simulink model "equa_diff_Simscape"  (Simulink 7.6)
settings: Solver=ode15s  StartTime=0.0  StopTime=30  RelTol=1e-3
InitFcn:
  | w0=0.5; z=sqrt(2)/2;
StopFcn:
  | close all
  | load equa_diff_RLC.mat
  | plot(x(1,:),x(2,:),x(1,:),x(3,:))
  | grid
  | axis([0 30 0 1.2])
  | title('entrée et tension aux bornes de la capacité - RLC')
  | xlabel('temps')
libraries: fl_lib x6, nesl_utility x3

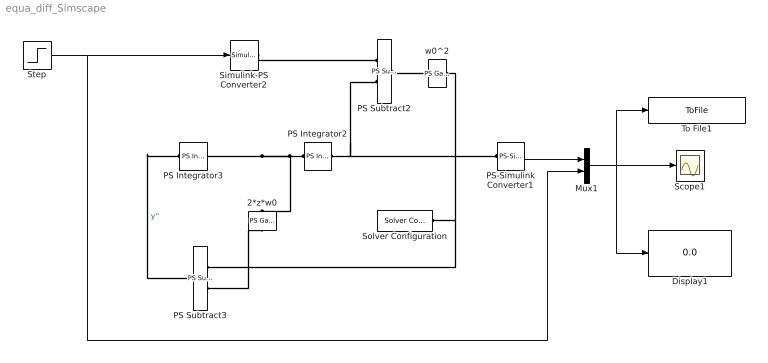
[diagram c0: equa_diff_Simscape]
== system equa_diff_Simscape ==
  2*z*w0 : fl_lib/Physical Signals/Functions/PS Gain  DialogController=NetworkEngine.DynNeDlgSource  SystemSampleTime=-1  gain=2*z*w0  LocalVarLogging=[]
  Display1 : Display
  Mux1 : Mux  Inputs=2
  PS Integrator2 : fl_lib/Physical Signals/Linear Operators/PS Integrator  DialogController=NetworkEngine.DynNeDlgSource  SystemSampleTime=-1  x0=0  x_Log=off  LocalVarNames=|x  LocalVarDescs=|x  LocalVarLogging=0
  PS Integrator3 : fl_lib/Physical Signals/Linear Operators/PS Integrator  DialogController=NetworkEngine.DynNeDlgSource  SystemSampleTime=-1  x0=0  x_Log=off  LocalVarNames=|x  LocalVarDescs=|x  LocalVarLogging=0
  PS Subtract2 : fl_lib/Physical Signals/Functions/PS Subtract  DialogController=NetworkEngine.DynNeDlgSource  SystemSampleTime=-1  LocalVarLogging=[]
  PS Subtract3 : fl_lib/Physical Signals/Functions/PS Subtract  DialogController=NetworkEngine.DynNeDlgSource  SystemSampleTime=-1  LocalVarLogging=[]
  PS-Simulink Converter1 : nesl_utility/PS-Simulink Converter  DialogController=NetworkEngine.DynNeUtilDlgSource  SystemSampleTime=-1  PhysicalDomain=network_engine_domain  LeftPortType=input  RightPortType=output  SubClassName=ps_output  Unit=1  AffineConversion=off
  Scope1 : Scope
  Simulink-PS Converter2 : nesl_utility/Simulink-PS Converter  DialogController=NetworkEngine.DynNeUtilDlgSource  SystemSampleTime=-1  PhysicalDomain=network_engine_domain  LeftPortType=input  RightPortType=output  SubClassName=ps_input  Unit=1  AffineConversion=off  InputFilterTimeConstant=.001  UdotUserProvided=0
  Solver Configuration : nesl_utility/Solver Configuration  DialogController=NetworkEngine.DynNeUtilDlgSource  SystemSampleTime=-1  PhysicalDomain=network_engine_domain  LeftPortType=input  RightPortType=generic  SubClassName=solver  Accelerate=off  Profile=off  ResidualTolerance=1e-9  MaxNonlinIter=3  MaxModeIter=2  DoFixedCost=off  UseLocalSampling=off  DoDC=off  LinearAlgebra=Sparse  LocalSolverSampleTime=.001  LocalSolverChoice=NE_BACKWARD_EULER_ADVANCER  UseLocalSolver=off
  Step : Step  Time=5  SampleTime=0
  To File1 : ToFile  Filename=equa_diff_RLC  MatrixName=x
  w0^2 : fl_lib/Physical Signals/Functions/PS Gain  DialogController=NetworkEngine.DynNeDlgSource  SystemSampleTime=-1  gain=w0^2  LocalVarLogging=[]
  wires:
  Mux1/1 -> Scope1/1, Display1/1, To File1/1
  PS-Simulink Converter1/1 -> Mux1/1
  Step/1 -> Mux1/2, Simulink-PS Converter2/1
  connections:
  Simulink-PS Converter2/RConn1 -- PS Subtract2/LConn1
  PS Subtract2/RConn1 -- w0^2/LConn1
  Solver Configuration/RConn1 -- w0^2/RConn1 -- PS Subtract3/LConn1
  PS Integrator2/RConn1 -- PS Subtract2/LConn2 -- PS-Simulink Converter1/LConn1
  PS Subtract3/RConn1 -- PS Integrator3/LConn1  "y''"
  PS Integrator2/LConn1 -- PS Integrator3/RConn1 -- 2*z*w0/LConn1
  PS Subtract3/LConn2 -- 2*z*w0/RConn1
